(* Logix 5000 DataType export Exlar_Control; software revision 32.02 *)

TYPE Exlar_Control :   // Tritex II Control
STRUCT
   EnableOutputs : INT;   // EnableOutputs
   InputEventsMode : INT;   // 4316
   InputEventsModeLevel : INT;   // 4318
   InputEventsMotion : INT;   // 4317
   HostCommandControlMode : INT;   // 4303
   HostPosition_low : INT;   // 4304
   HostPosition_high : INT;
   HostVelocity_low : INT;   // 4306
   HostVelocity_high : INT;
   HostAcceleration_low : INT;   // 4308
   HostAcceleration_high : INT;
   HostCurrent : INT;   // 4310
   InputEventsMoveEdge : INT;   // 4319
   JogSlowVelocity_low : INT;   // 6022
   JogSlowVelocity_high : INT;
   JogAcceleration_low : INT;   // 6026
   JogAcceleration_high : INT;
   MoveOption : INT;   // 6100
   MoveCurrentLimit : INT;   // 6101
   MoveAcceleration_low : INT;   // 6102
   MoveAcceleration_high : INT;
   MoveDeceleration_low : INT;   // 6500
   MoveDeceleration_high : INT;
   MovePrimaryOption : INT;   // 6106
   spare : INT;   // spare
   MovePrimaryPosition_low : INT;   // 6108
   MovePrimaryPosition_high : INT;
   MovePrimaryVelocity_low : INT;   // 6110
   MovePrimaryVelocity_high : INT;
   MoveSecondaryOption : INT;   // 6112
   spare2 : INT;   // spare
   MoveSecondaryPosition_low : INT;   // 6114
   MoveSecondaryPosition_high : INT;
   MoveSecondaryVelocity_low : INT;   // 6116
   MoveSecondaryVelocity_high : INT;
END_STRUCT
END_TYPE
